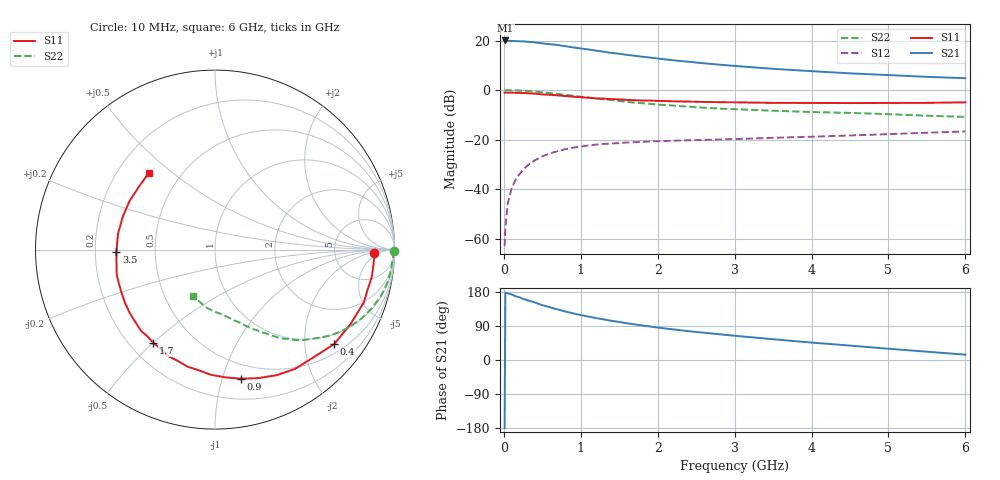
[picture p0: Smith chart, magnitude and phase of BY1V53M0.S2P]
! SIEMENS Small Signal Semiconductors
! BFY420
! Si NPN RF SIEGET Grounded Emitter Transistor in MICRO-X
! VCE = 1.5 V  IC = 3 mA
! Common Emitter S-Parameters:  October  1996
# GHz  S  MA  R  50
!  f  S11  S21  S12  S22
! GHz  MAG  ANG  MAG  ANG  MAG  ANG  MAG  ANG
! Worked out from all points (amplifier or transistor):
!   36 points, 10 MHz to 6 GHz, reference 50 ohm
!   highest |S21| = 20.0 dB at 20 MHz (marker M1)
!   |S21| within 3 dB of that: start of sweep to 945.2 MHz
!   unconditionally stable (mu >= 1): 3.601 GHz to end of sweep
!   at 250 MHz: K = 0.09, MSG = 25.9 dB, |S12| = -32.2 dB
!   at 1.4 GHz: K = 0.39, MSG = 18.3 dB, |S12| = -21.6 dB
!   at 6 GHz: K = 1.21, MAG = 8.0 dB, |S12| = -16.7 dB
!   S11 on the Smith chart (normalised r, x): 10 MHz: 16, -3; 400 MHz: 0.72, -2.70; 900 MHz: 0.37, -1.15; 1.7 GHz: 0.29, -0.50; 3.5 GHz: 0.29, -0.01; 6 GHz: 0.33, +0.41
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0.01  0.8882 -1.3  9.991 -179.8  0.0007 94.3  0.9953 -0.5
0.02  0.8887 -2.3  10.03 178.2  0.0017 99.6  0.9911 -1.0
0.05  0.8873 -5.0  9.822 175.8  0.005 86.0  0.9924 -2.6
0.1  0.8869 -10.0  9.801 173.0  0.0101 83.4  0.9883 -5.3
0.15  0.8794 -14.5  9.736 168.4  0.0151 81.5  0.9838 -8.1
0.2  0.8798 -19.6  9.668 165.6  0.0197 79.2  0.9785 -10.6
0.3  0.8616 -29.0  9.479 158.0  0.0293 74.5  0.9595 -15.7
0.4  0.8475 -38.4  9.177 152.0  0.0378 68.2  0.932 -20.7
0.5  0.8142 -47.2  8.747 144.7  0.0455 64.3  0.9023 -25.1
0.6  0.8005 -56.1  8.442 139.1  0.0526 59.7  0.8692 -29.4
0.7  0.7796 -63.8  8.096 133.4  0.0582 55.9  0.8344 -33.3
0.9  0.7339 -78.6  7.262 123.0  0.0685 48.4  0.7636 -39.9
1.1  0.6984 -91.7  6.6 114.5  0.0759 43.2  0.7033 -45.7
1.4  0.6529 -108.9  5.615 103.4  0.0831 36.8  0.6256 -52.5
1.7  0.623 -123.6  4.927 94.0  0.0882 32.3  0.5549 -58.0
2  0.603 -136.2  4.328 85.6  0.0923 29.0  0.5085 -62.3
2.2  0.592 -143.2  3.992 80.8  0.0945 27.1  0.4849 -65.2
2.8  0.5676 -161.0  3.255 68.0  0.1004 23.9  0.4227 -72.3
3.5  0.5499 -178.4  2.682 54.8  0.1082 21.6  0.3811 -79.6
4.5  0.5455 160.3  2.17 38.0  0.1206 18.7  0.3449 -91.1
5.5  0.5505 139.9  1.846 21.9  0.1369 15.1  0.3022 -106.6
6  0.5637 131.0  1.731 14.1  0.1457 13.1  0.286 -115.9
